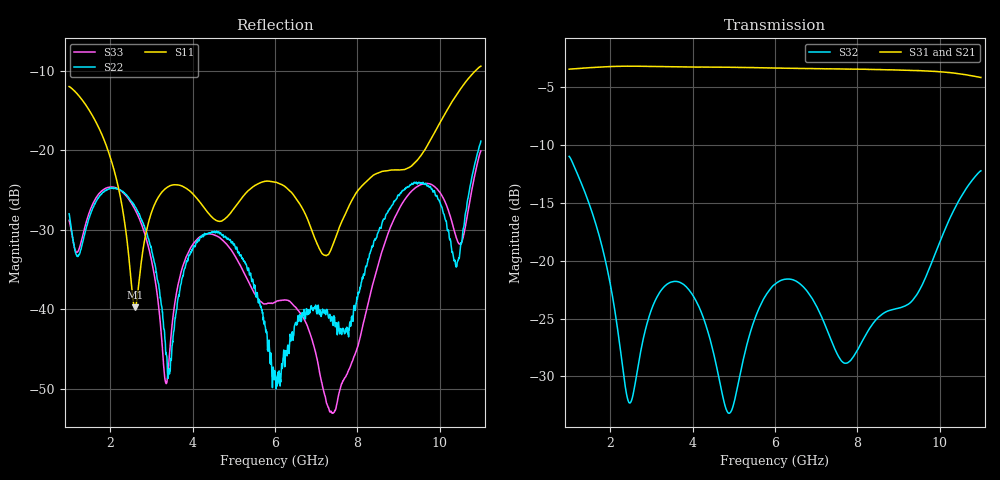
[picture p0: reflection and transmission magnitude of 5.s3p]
!The following data was pulled from an Agilent PNA
!This sNp file was generated from the data in the RF Test software
!NOTE:  Smoothing/Math/Corrections applied on any given trace ARE included in the data saved here
# MHz S dB R 50
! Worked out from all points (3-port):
!   1601 points, 1 GHz to 11 GHz, reference 50 ohm
!   strongest paths, dB at 1 GHz, 3.5 GHz, 6 GHz, 8.5 GHz, 11 GHz:
!     S31: -3.4, -3.2, -3.3, -3.5, -4.1
!     S21: -3.4, -3.2, -3.3, -3.4, -4.1
!     S32: -11.0, -21.8, -22.0, -24.9, -12.2
!   lowest |S11| = -39.8 dB at 2.6 GHz (marker M1), VSWR 1.02, Z = 49.2 + j0.611 ohm
!   |S11| at or under -10 dB: start of sweep to 10.87 GHz
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1000  -12.01 131.6  -3.42 -64.7  -3.42 -63.9
      -3.43 -63.9  -28.00 16.5  -10.97 -86.5
      -3.42 -64.0  -10.97 -86.5  -28.82 10.2
2600  -39.78 142.7  -3.18 -170.2  -3.17 -170.5
      -3.17 -170.2  -27.11 124.9  -30.71 -64.3
      -3.16 -170.5  -30.70 -64.1  -27.46 127.5
3356.25  -24.77 -170.0  -3.21 139.0  -3.21 138.5
         -3.21 139.0  -45.44 114.6  -22.10 -72.0
         -3.20 138.5  -22.09 -72.0  -49.35 160.6
4175  -26.53 175.1  -3.25 83.9  -3.24 83.3
      -3.24 83.9  -31.09 177.3  -24.17 -113.2
      -3.23 83.3  -24.16 -113.2  -30.90 -175.2
4893.75  -28.08 -148.9  -3.27 35.0  -3.26 34.3
         -3.27 35.0  -31.25 123.8  -33.21 -86.7
         -3.26 34.3  -33.20 -86.9  -32.25 125.0
6000  -24.01 -155.7  -3.33 -41.2  -3.32 -42.1
      -3.33 -41.2  -47.74 -21.1  -22.02 -82.3
      -3.33 -42.1  -22.01 -82.3  -39.11 -40.0
7956.25  -25.49 -86.7  -3.42 -179.1  -3.42 179.7
         -3.42 -179.2  -39.93 158.3  -28.02 -103.2
         -3.42 179.6  -28.01 -103.2  -45.47 -135.9
9325  -21.95 -82.7  -3.51 80.8  -3.53 79.4
      -3.51 80.8  -24.16 68.7  -23.49 -101.8
      -3.53 79.3  -23.49 -101.7  -25.12 56.5
10412.5  -13.00 -81.2  -3.76 -1.7  -3.79 -3.3
         -3.76 -1.7  -34.63 -93.9  -15.14 -115.1
         -3.79 -3.3  -15.14 -115.1  -31.15 -77.3
11000  -9.45 -106.8  -4.10 -45.6  -4.15 -48.5
       -4.11 -46.7  -18.86 141.4  -12.23 -144.3
       -4.14 -48.5  -12.21 -144.3  -20.10 140.1
